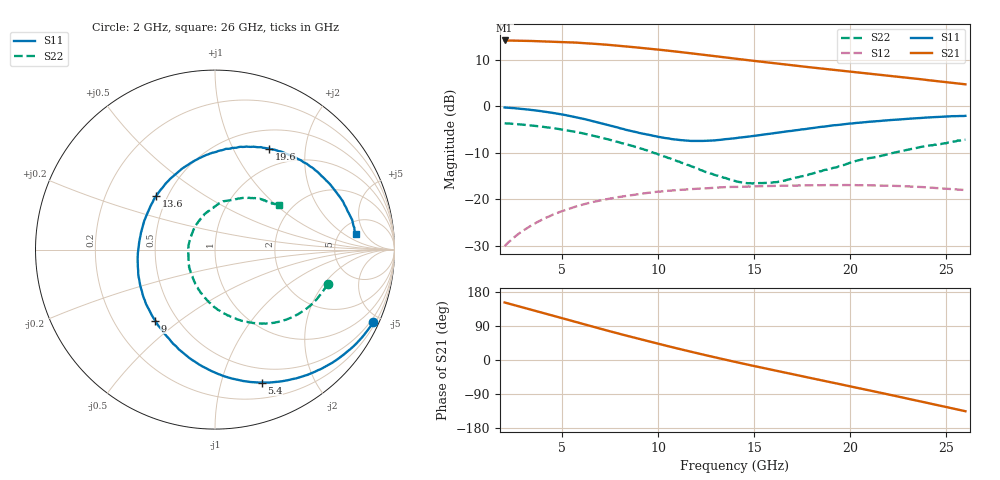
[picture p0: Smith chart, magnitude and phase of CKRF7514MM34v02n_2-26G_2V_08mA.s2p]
! CHUO DENSHI KOGYO Co.,Ltd.
! 22. July 2016
! CKRF7514MM34
! N-channel HJ-FET
! Vds = 2 V Id = 8 mA
# Hz S  MA  R 50
!	f	S11	S21	S12	S22
!	Hz	MAG	ANG	MAG	ANG	MAG	ANG	MAG	ANG
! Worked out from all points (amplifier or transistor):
!   241 points, 2 GHz to 26 GHz, reference 50 ohm
!   highest |S21| = 14.1 dB at 2 GHz (marker M1)
!   |S21| within 3 dB of that: start of sweep to 12.19 GHz
!   unconditionally stable (mu >= 1): 12.47 GHz to 19.71 GHz
!   at 6 GHz: K = 0.61, MSG = 17.4 dB, |S12| = -21.2 dB
!   at 14 GHz: K = 1.03, MAG = 12.7 dB, |S12| = -17.4 dB
!   at 26 GHz: K = 0.83, MSG = 11.4 dB, |S12| = -18.0 dB
!   lowest NFmin = 0.33 dB at 10 GHz
!   S11 on the Smith chart (normalised r, x): 2 GHz: 0.33, -4.53; 5.4 GHz: 0.35, -1.35; 9 GHz: 0.38, -0.41; 13.6 GHz: 0.43, +0.33; 19.6 GHz: 0.74, +1.40; 26 GHz: 6.96, +3.19
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2e9  0.9698 -24.7  5.094 151.8  0.03131 73.3  0.6558 -17.0
2.9e9  0.9364 -36.3  5.05 139.4  0.04516 66.2  0.6348 -24.6
3.7e9  0.8955 -46.9  5.009 128.3  0.05682 59.6  0.6112 -31.7
4.6e9  0.841 -59.1  4.94 115.8  0.06932 52.3  0.5786 -39.8
5.4e9  0.7858 -70.6  4.865 104.6  0.07971 45.8  0.5428 -47.2
6e9  0.7398 -79.4  4.796 96.3  0.08696 41.1  0.5152 -53.0
6.6e9  0.6918 -88.8  4.706 87.9  0.09345 36.1  0.4823 -58.6
7.4e9  0.6277 -101.8  4.568 76.9  0.1009 29.9  0.4389 -66.3
8.1e9  0.5744 -113.9  4.435 67.5  0.1066 24.8  0.4007 -73.2
9e9  0.5168 -130.0  4.263 55.8  0.1138 18.8  0.3564 -82.7
1e10  0.469 -150.2  4.066 42.9  0.1208 11.8  0.3037 -94.4
1.08e10  0.4411 -166.9  3.897 32.9  0.1246 6.4  0.2661 -104.0
1.17e10  0.4238 174.1  3.709 21.9  0.1287 0.7  0.2269 -117.1
1.26e10  0.4254 155.7  3.524 11.2  0.1315 -4.7  0.1933 -132.2
1.36e10  0.444 137.2  3.325 -0.3  0.1354 -10.9  0.1666 -152.1
1.4e10  0.4523 130.2  3.249 -4.8  0.1357 -13.5  0.1574 -160.0
1.59e10  0.5091 102.6  2.922 -25.8  0.139 -24.2  0.1508 156.4
1.8e10  0.5808 77.9  2.609 -48.2  0.1415 -36.1  0.1876 115.3
1.96e10  0.6378 61.9  2.404 -65.3  0.142 -45.8  0.2322 93.5
2.2e10  0.7081 40.3  2.126 -91.0  0.1398 -61.5  0.3061 66.8
2.4e10  0.7564 22.4  1.913 -113.1  0.134 -76.3  0.3742 49.1
2.6e10  0.7884 6.3  1.72 -135.2  0.1256 -91.9  0.4363 35.0
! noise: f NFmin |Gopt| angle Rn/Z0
1e+10  0.33  0.471  101.4  0.07
1.05e+10  0.35  0.448  110.2  0.06
1.1e+10  0.36  0.42  119.8  0.05
1.15e+10  0.38  0.39  129  0.05
1.2e+10  0.41  0.363  140.7  0.04
1.25e+10  0.42  0.343  154.1  0.04
1.3e+10  0.44  0.326  165.6  0.04
1.35e+10  0.46  0.321  179.9  0.03
1.4e+10  0.5  0.326  -166.5  0.04
1.5e+10  0.54  0.346  -143.7  0.04
